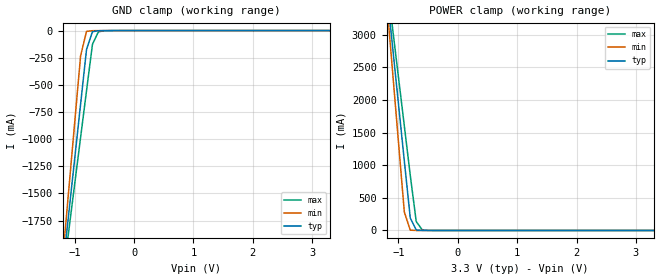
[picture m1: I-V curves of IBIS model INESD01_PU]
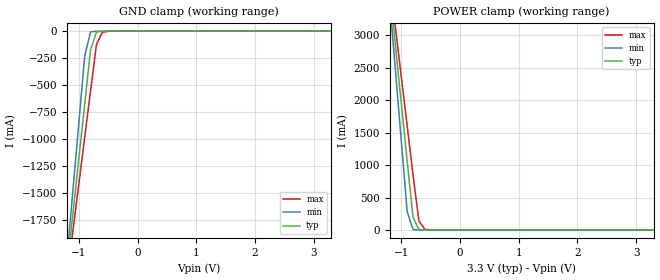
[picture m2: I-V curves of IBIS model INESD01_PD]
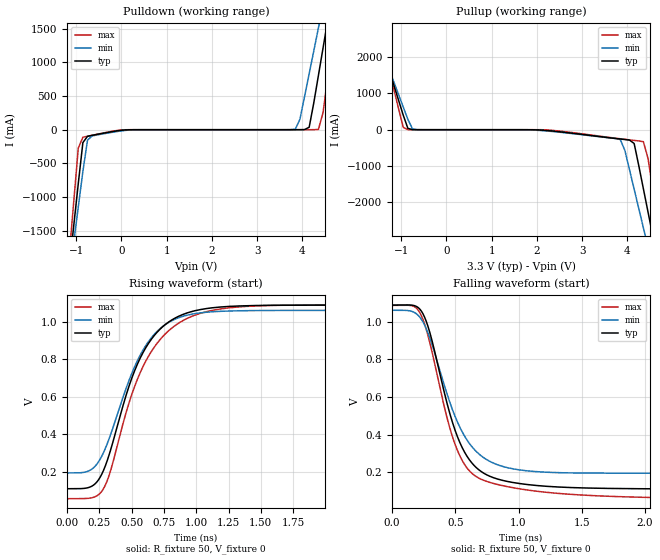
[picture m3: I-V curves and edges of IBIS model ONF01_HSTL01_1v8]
|   This file is an IBIS representation of the   |
|   Integrated Device Technology, Inc.   |
|   ICS8525   |
|   Low Skew 1 to 4 LVCMOS to LVHSTL Fanout Buffer   |
[IBIS Ver]   4.1
[File name]   8525_3v3.ibs
[File Rev]   2.0
[Date]   2 Sep 2009 | Last modified
|   12 Dec 2000 | Generated
[Source]   Originated at Integrated Device Technology, Inc.
[Disclaimer]
IDT hereby grants the user of this IBIS model a non-exclusive,
nontransferable license to use this IBIS model under the following terms.
Before using this IBIS model, the user should read this license.
If the user does not accept these terms,  the IBIS model should be
returned to IDT within 30 days.
   The user is granted this license only to use the IBIS model and
is not granted rights to sell, load, rent, lease or license the IBIS
model in whole or in part, or in modified form to anyone other than
user. User may modify the IBIS model to suit its specific
applications but rights to derivative works and such modifications
shall belong to IDT.
   This IBIS model is provided on an "AS IS" basis and IDT makes
absolutely no warranty with respect to the information contained
herein. IDT DISCLAIMS AND CUSTOMER WAIVES ALL WARRANTIES, EXPRESS
OR IMPLIED, INCLUDING WARRANTIES OF MERCHANTABILITY OR FITNESS FOR
A PARTICULAR PURPOSE. The entire risk as to quality and performance
is with the Customer. ACCORDINGLY, IN NO EVENT SHALL THE COMPANY BE
LIABLE FOR ANY DAMAGES, WHETHER IN CONTRACT OR TORT,INCLUDING ANY
LOST PROFITS OR OTHER INCIDENTAL, CONSEQUENTIAL, EXEMPLARY, OR
PUNITIVE DAMAGES ARISING OUT OF THE USE OR APPLICATION OF THE IBIS
model provided in this package. Further, IDT reserves the right to
make changes without notice to any product herein to improve
reliability, function, or design. IDT does not convey any license
under patent rights or any other intellectual property rights,
including those of third parties.
   IDT is not obligated to provide maintenance or support
for the licensed IBIS model.
[Copyright]   Copyright 2005 by Integrated Device Technology, Inc.
[Component]   ICS8525
[Manufacturer] Integrated Device Technology, Inc.
[Package]
|TSSOP 20 Lead
|   typ   min   max
R_pkg   51.85m   41.1m   62.6m
L_pkg   1.568nH   0.734nH   2.401nH
C_pkg   0.221pF   0.068pF   0.373pF
[Pin] signal_name   model_name   R_pin   L_pin   C_pin
1   GND   GND   62.6m   2.401n   0.373p
2   CLK_EN   INESD01_PU   57.23m   1.985n   0.297p
3   CLK_SEL   INESD01_PD   51.85m   1.568n   0.221p
4   CLK0   INESD01_PD   46.78m   1.151n   0.145p
5   NC   NC   41.1m   0.734n   0.068p
6   CLK1   INESD01_PD   41.1m   0.734n   0.068p
7   NC   NC   46.78m   1.151n   0.145p
8   NC   NC   51.85m   1.568n   0.221p
9   NC   NC   57.23m   1.985n   0.297p
10   VDD   POWER   62.6m   2.401n   0.373p
11   nQ3   ONF01_HSTL01_1v8   62.6m   2.401n   0.373p
12   Q3   ONF01_HSTL01_1v8   57.23m   1.985n   0.297p
13   VDDO   POWER   51.85m   1.568n   0.221p
14   nQ2   ONF01_HSTL01_1v8   46.78m   1.151n   0.145p
15   Q2   ONF01_HSTL01_1v8   41.1m   0.734n   0.068p
16   nQ1   ONF01_HSTL01_1v8   41.1m   0.734n   0.068p
17   Q1   ONF01_HSTL01_1v8   46.78m   1.151n   0.145p
18   VDDO   POWER   51.85m   1.568n   0.221p
19   nQ0   ONF01_HSTL01_1v8   57.23m   1.985n   0.297p
20   Q0   ONF01_HSTL01_1v8   62.6m   2.401n   0.373p
[Diff Pin]  inv_pin  vdiff tdelay_typ tdelay_min  tdelay_max
12   11   NA   0  0  0
15   14   NA   0  0  0
17   16   NA   0  0  0
20   19   NA   0  0  0
| Models and submodels in the file (3): INESD01_PU (Input), INESD01_PD (Input), ONF01_HSTL01_1v8 (Output)
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[Model]   INESD01_PU
Model_type   Input
Polarity   Non-Inverting
Vinl = 0.8V
Vinh = 2.0V
|   typ   min   max
C_comp   2pF   1.5pF   2.5pF
|   typ   min   max
[Voltage range]  3.3V   3.15V   3.45V
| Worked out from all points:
|   GND clamp passes 1 mA (typ) near -0.55 V on its own axis
|   POWER clamp passes 1 mA (typ) near -0.61 V on its own axis
[GND_clamp]
|Voltage   I(typ)   I(min)   I(max)
-3.3V     -12.83A    -15.14A    -11.37A
-1.2V     -2.195A    -2.092A    -2.281A
-1.1V     -1.689A    -1.472A    -1.849A
-900mV    -678.5mA   -232.7mA   -984.8mA
-800mV    -174mA     -7.237mA   -553.3mA
-700mV    -9.767mA   -1.114mA   -126.1mA
-600mV    -1.7mA     -240.1uA   -11.15mA
-300mV    -81.66uA   -67.79uA   -163.4uA
3.3V      1.866nA    1.113pA    239.1nA
[POWER_clamp]
|Voltage   I(typ)   I(min)   I(max)
-3.3V     22.38A     26.45A     19.82A
-1.2V     3.723A     3.545A     3.874A
-1.1V     2.836A     2.457A     3.116A
-1V       1.949A     1.369A     2.358A
-900mV    1.063A     281mA      1.601A
-800mV    191.5mA    5.012mA    843.9mA
-700mV    8.032mA    142.2uA    138.3mA
-600mV    607uA      17.63uA    10.62mA
-400mV    16.32uA    7.545uA    335.9uA
3.3V      -71.13uA   -62.11uA   -78.26uA
[Model]   INESD01_PD
Model_type   Input
Polarity   Non-Inverting
Vinl = 0.80V
Vinh = 2.0V
|   typ   min   max
C_comp   2pF   1.5pF   2.5pF
|   typ   min   max
[Voltage range]  3.3V   3.15V   3.45V
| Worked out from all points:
|   GND clamp passes 1 mA (typ) near -0.55 V on its own axis
|   POWER clamp passes 1 mA (typ) near -0.60 V on its own axis
[GND_clamp]
|Voltage I(typ)   I(min)   I(max)
-3.3V     -12.83A    -15.14A    -11.37A
-1.2V     -2.195A    -2.092A    -2.281A
-1.1V     -1.689A    -1.472A    -1.849A
-900mV    -678.5mA   -232.6mA   -984.8mA
-800mV    -173.9mA   -7.175mA   -553.2mA
-700mV    -9.696mA   -1.052mA   -126mA
-600mV    -1.629mA   -178uA     -11.07mA
-300mV    -10.53uA   -5.678uA   -86.08uA
3.3V      71.13uA    62.11uA    77.58uA
[POWER_clamp]
|Voltage   I(typ)   I(min)   I(max)
-3.3V     22.38A     26.45A     19.82A
-1.2V     3.723A     3.545A     3.874A
-1.1V     2.836A     2.457A     3.116A
-1V       1.949A     1.369A     2.358A
-900mV    1.063A     281.1mA    1.601A
-800mV    191.6mA    5.074mA    844mA
-700mV    8.104mA    204.3uA    138.4mA
-600mV    678.1uA    79.74uA    10.7mA
-400mV    87.44uA    69.65uA    413.2uA
3.3V      -3.041nA   -425fA     -919.9nA
[Model]   ONF01_HSTL01_1v8
|3.3V core, 1.8V output supply
Model_type  Output
Polarity   Non-Inverting
Vmeas = .6
Rref = 50
Cref = 0
Vref = 0
|Variable  typ   min   max
C_comp   2p   1.5p   2.5p
[Voltage Range]   3.3   3.135   3.465
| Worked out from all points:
|   slope of the pulldown table from 0 to 0.495 V, typ, clamps not added: 54.9 ohm
|   rising waveform, R_fixture 50, V_fixture 0: 20-80 % time 306ps typ, 302ps min, 333ps max; typ from 0.111 V to 1.09 V
|   falling waveform, R_fixture 50, V_fixture 0: 20-80 % time 255ps typ, 284ps min, 252ps max; typ from 1.09 V to 0.111 V
| Open source, no load
|  Voltage   I(typ)   I(min)   I(max)
[Pulldown]
-3.3V     -15.42A    -13.35A    -18.91A
-1.157V   -2.072A    -2.21A     -1.894A
-1.055V   -1.436A    -1.68A     -1.084A
-952.6mV  -800.4mA   -1.149A    -274.1mA
-850.5mV  -191.4mA   -618.4mA   -111.9mA
-544.3mV  -70.23mA   -78.22mA   -68.72mA
3.844V    27.09uA    7.698mA    3.013nA
4.151V    36.63mA    830.7mA    49.54uA
4.355V    803.8mA    1.508A     4.53mA
4.559V    1.617A     2.187A     770.5mA
4.763V    2.432A     2.867A     1.809A
6.6V      9.786A     9.002A     11.19A
[Pullup]
-3.3V     9.786A     8.45A      12.03A
-1.565V   2.839A     2.657A     3.17A
-1.463V   2.432A     2.317A     2.65A
-952.6mV  398mA      622.1mA    64.71mA
-850.5mV  36.63mA    284.2mA    1.532mA
-646.4mV  229.4uA    1.613mA    19.07uA
3.844V    -256mA     -270.5mA   -249.6mA
4.151V    -379.9mA   -1.636A    -294.5mA
4.355V    -1.626A    -2.699A    -329.8mA
4.559V    -2.898A    -3.761A    -1.602A
4.763V    -4.17A     -4.823A    -3.222A
6.6V      -15.62A    -14.38A    -17.8A
[Ramp]
|   typ   min   max
dV/dt_r   0.782/0.488n   0.693/0.472n   0.826/0.535n
dV/dt_f   0.783/0.418n   0.693/0.453n   0.822/0.447n
R_load =   50.0000
[Rising Waveform]
R_fixture = 50
V_fixture = 0
C_fixture = 0.0p
| Time   typ   min   max
0s        110.9mV    195.1mV    57.72mV
173.6ps   118.9mV    207.8mV    60.43mV
275.9ps   199mV      294.5mV    104.4mV
334.8ps   312.4mV    395.2mV    202.7mV
480.5ps   659.8mV    690.1mV    570.6mV
579.7ps   826mV      840.3mV    750.2mV
728.5ps   967.2mV    969.3mV    912.9mV
917.6ps   1.045V     1.034V     1.015V
1.423ns   1.087V     1.06V      1.084V
2.998ns   1.089V     1.062V     1.089V
[Falling Waveform]
R_fixture = 50
V_fixture = 0
C_fixture = 0.0p
| Time   typ   min   max
0s        1.089V     1.062V     1.088V
170.5ps   1.087V     1.052V     1.083V
244.9ps   1.042V     999.2mV    1.011V
303.8ps   931.1mV    904.4mV    875.3mV
421.6ps   601.8mV    644.6mV    525.1mV
492.9ps   434.4mV    506.4mV    359mV
582.8ps   296.3mV    382.4mV    232.4mV
691.3ps   210.9mV    295.1mV    167.5mV
1.163ns   128.8mV    202.7mV    97.96mV
2.998ns   111.1mV    195.1mV    59.79mV
